(* Logix 5000 AddOnInstructionDefinition export Bronkhorst_FF_Basic_REAL_Input; software revision 37.00 *)

ADD_ON_INSTRUCTION Bronkhorst_FF_Basic_REAL_Input   (* revision 1.0, vendor Bronkhorst High-Tech B.V. *)
// Extract data from the FLEXI-FLOW Basic REAL input connection (in to controller from device)
VAR_IN_OUT
   DataIn : SINT[13]; {required}
END_VAR
VAR_OUTPUT
   Status : USINT; {visible}
   Measure : REAL; {visible}
   Pressure_Inlet : REAL; {visible}
   Pressure_Outlet : REAL; {visible}
END_VAR

ROUTINE Logic   (* structured text *)
   Status := DataIn[0];
   COP(DataIn[1], Measure, 1);
   COP(DataIn[5], Pressure_Inlet, 1);
   COP(DataIn[9], Pressure_Outlet, 1);
END_ROUTINE
END_ADD_ON_INSTRUCTION

ADD_ON_INSTRUCTION Bronkhorst_FF_Basic_REAL_Output   (* revision 1.0, vendor Bronkhorst High-Tech B.V. *)
// Fill data for the FLEXI-FLOW Basic Real output connection (out from controller to device)
VAR_IN_OUT
   DataOut : SINT[12]; {required}
END_VAR
VAR_INPUT
   Setpoint : REAL; {visible}
   Pressure_Inlet_Setpoint : REAL; {visible}
   Pressure_Outlet_Setpoint : REAL; {visible}
END_VAR

ROUTINE Logic   (* structured text *)
   COP(Setpoint, DataOut[0], 4);
   COP(Pressure_Inlet_Setpoint, DataOut[4], 4);
   COP(Pressure_Outlet_Setpoint, DataOut[8], 4);
END_ROUTINE
END_ADD_ON_INSTRUCTION
